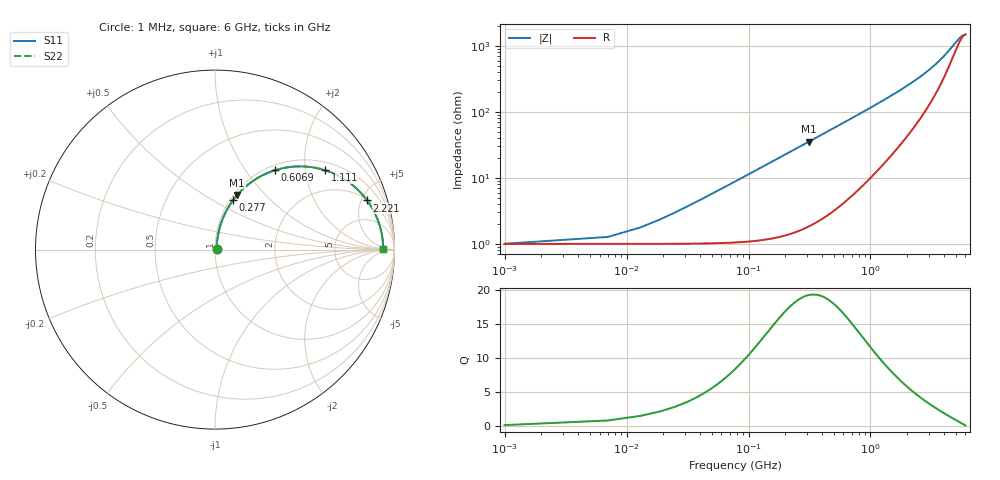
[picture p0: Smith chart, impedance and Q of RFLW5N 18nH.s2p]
!Vishay Electro-Films
!RFLW5N1800B - 18 nH Spiral Inductor on Quartz
!Measured in series configuration
!May 2011
# GHz S MA R 50
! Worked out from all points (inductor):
!   1001 points, 1 MHz to 6 GHz, reference 50 ohm
!   read as one part in series: L = 18 nH near 31 MHz
!   highest Q = 19.2 at 312.9 MHz (marker M1), where L = 18 nH
!   S11 on the Smith chart (normalised r, x): 1 MHz: 1.02, +0.00; 277 MHz: 1.03, +0.63; 606.9 MHz: 1.08, +1.38; 1.111 GHz: 1.24, +2.58; 2.221 GHz: 2.10, +5.58; 6 GHz: 31, +2
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0.001  0.009958 6.4  0.9901 -0.1  0.9901 -0.1  0.009958 6.4
0.018997  0.02344 63.7  0.9899 -1.2  0.9899 -1.2  0.02344 63.7
0.048992  0.05562 76.4  0.9884 -3.1  0.9884 -3.1  0.05562 76.4
0.066989  0.07538 77.9  0.987 -4.3  0.987 -4.3  0.07538 77.9
0.090985  0.1017 78.2  0.9843 -5.8  0.9843 -5.8  0.1017 78.2
0.126979  0.1409 77.4  0.979 -8.1  0.979 -8.1  0.1409 77.4
0.168972  0.1857 75.6  0.9706 -10.7  0.9706 -10.7  0.1857 75.6
0.276954  0.2949 69.8  0.94 -17.1  0.94 -17.1  0.2949 69.8
0.312948  0.3289 67.8  0.9274 -19.2  0.9274 -19.2  0.3289 67.8
0.444926  0.4416 60.8  0.8738 -26.2  0.8738 -26.2  0.4416 60.8
0.606899  0.5536 53.0  0.7998 -33.5  0.7998 -33.5  0.5536 53.0
0.786869  0.6475 45.7  0.7171 -40.2  0.7171 -40.2  0.6475 45.7
1.00283  0.7274 38.6  0.6262 -46.4  0.6262 -46.4  0.7274 38.6
1.11082  0.7574 35.6  0.5854 -48.9  0.5854 -48.9  0.7574 35.6
1.50675  0.8309 27.2  0.4614 -55.5  0.4614 -55.5  0.8309 27.2
2.00467  0.8782 20.2  0.3505 -59.9  0.3505 -59.9  0.8782 20.2
2.22063  0.8908 17.9  0.3134 -60.9  0.3134 -60.9  0.8908 17.9
3.0005  0.9169 11.8  0.2137 -61.4  0.2137 -61.4  0.9169 11.8
4.00233  0.9307 6.7  0.1324 -55.1  0.1324 -55.1  0.9307 6.7
5.00417  0.9359 3.1  0.08244 -37.4  0.08244 -37.4  0.9359 3.1
5.54408  0.937 1.5  0.06765 -20.6  0.06765 -20.6  0.937 1.5
6  0.9373 0.2  0.06281 -3.3  0.06281 -3.3  0.9373 0.2
